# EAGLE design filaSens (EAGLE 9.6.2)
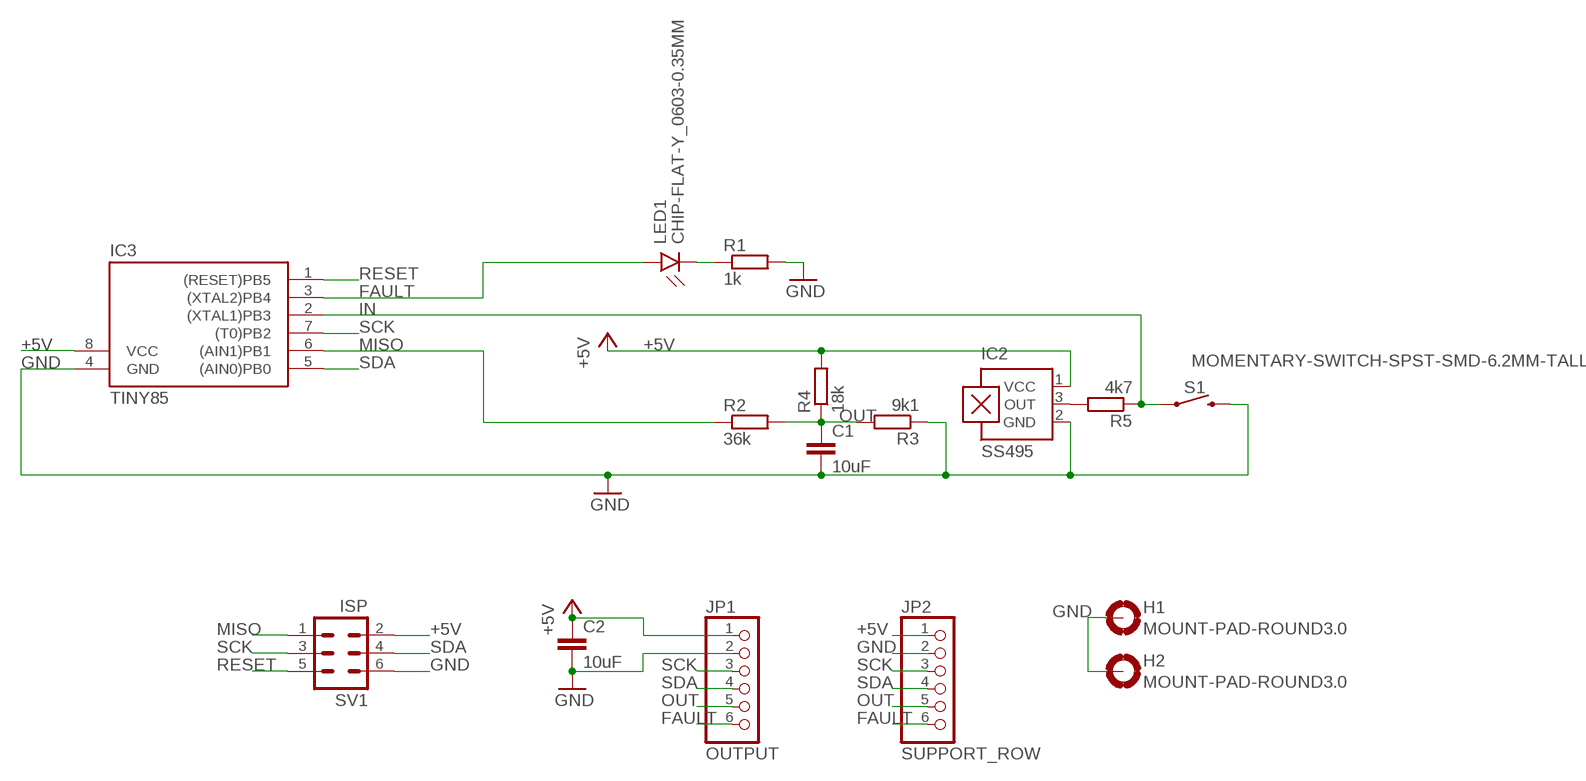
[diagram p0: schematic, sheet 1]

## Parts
C1  10uF  C-EUC0402  [C0402]
C2  10uF  C-EUC0402  [C0402]
H1  MOUNT-PAD-ROUND3.0  [3,0-PAD]
H2  MOUNT-PAD-ROUND3.0  [3,0-PAD]
IC2  SS495  A1302UA  [SIP3-UA]
IC3  TINY85  TINY10S  [SOIC8]
JP1  OUTPUT  PINHD-1X6  [1X06]
JP2  SUPPORT_ROW  PINHD-1X6  [1X06]
LED1  CHIP-FLAT-Y_0603-0.35MM  [LEDC1608X35N_FLAT-Y]
R1  1k  R-EU_R0402  [R0402]
R2  36k  R-EU_R0402  [R0402]
R3  9k1  R-EU_R0402  [R0402]
R4  18k  R-EU_R0402  [R0402]
R5  4k7  R-EU_R0402  [R0402]
S1  MOMENTARY-SWITCH-SPST-SMD-6.2MM-TALL  [TACTILE_SWITCH_SMD_6.2MM_TALL]
SV1  ISP  MA03-2  [MA03-2]

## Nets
+5V [power]: C2.1 IC2.1(VCC) IC3.8(VCC) JP1.1 JP2.1 R4.2 SV1.2
FAULT: IC3.3((XTAL2)PB4) JP1.6 JP2.6 LED1.A
GND [power]: C1.2 C2.2 H1.B3,0(MOUNT) H2.B3,0(MOUNT) IC2.2(GND) IC3.4(GND) JP1.2 JP2.2 R1.2 R3.1 S1.B2 SV1.6
IN: IC3.2((XTAL1)PB3) R5.1 S1.A2
MISO: IC3.6((AIN1)PB1) R2.1 SV1.1
N$1: IC2.3(OUT) R5.2
N$2: LED1.C R1.1
OUT: C1.1 JP1.5 JP2.5 R2.2 R3.2 R4.1
RESET: IC3.1((RESET)PB5) SV1.5
SCK: IC3.7((T0)PB2) JP1.3 JP2.3 SV1.3
SDA: IC3.5((AIN0)PB0) JP1.4 JP2.4 SV1.4

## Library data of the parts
C1 C2 = rcl:C-EU: CAPACITOR, European symbol; SPICEPREFIX: C
H1 H2 = holes:MOUNT-PAD-ROUND: MOUNTING PAD, round
IC2 = allegro:A13*?: Linear Hall Effect Sensor ICs Continuous-Time Ratiometric High-Temperature Operation Programmable Linear with Analog Output A1302 -Replacement- UGN3503 Source: http://www.allegromicro.com/en/Products/Part_Numbers/1301/1301.pdf http://www.allegromicro.com/en/Products/Part_Numbers/1321/1321.pdf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; MF: ALLEGRO MICROSYSTEMS, INC.; MPN: A1302EUA-T; OC_FARNELL: 1521708; OC_NEWARK: 31K6639
IC3 = atmel:TINY10: MICROCONTROLLER 1 Kbytes ROM; OC_FARNELL: unknown; OC_NEWARK: unknown
JP1 JP2 = pinhead:PINHD-1X6: PIN HEADER
LED1 = LED:CHIP-FLAT-Y; CATEGORY: LED; COLOR: YELLOW; DESCRIPTION: CHIP LED FLAT; SUB-CATEGORY: CHIP; TYPE: FLAT_TOP
R1-R5 = rcl:R-EU_: RESISTOR, European symbol; SPICEPREFIX: R
S1 = SparkFun-Switches:MOMENTARY-SWITCH-SPST: Momentary Switch (Pushbutton) - SPST; PROD_ID: SWCH-11966; SF_SKU: COM-12992
SV1 = con-lstb:MA03-2: PIN HEADER; OC_FARNELL: unknown; OC_NEWARK: unknown

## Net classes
0 default: width 0.254 mm
1 power: width 0.254 mm

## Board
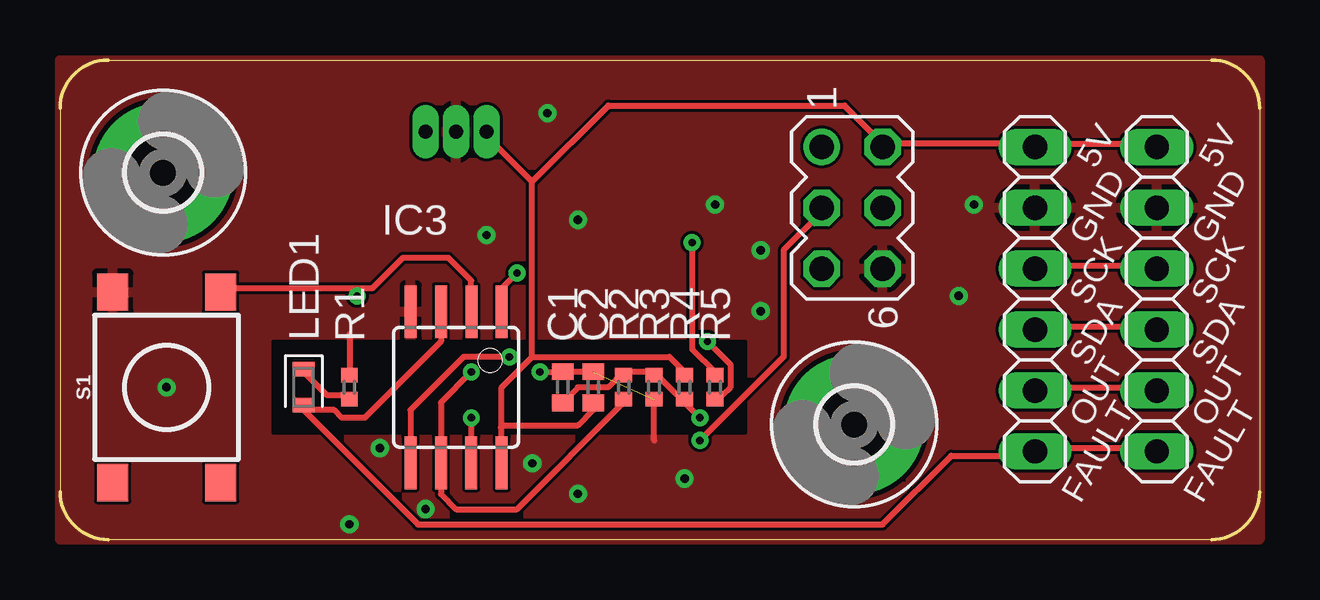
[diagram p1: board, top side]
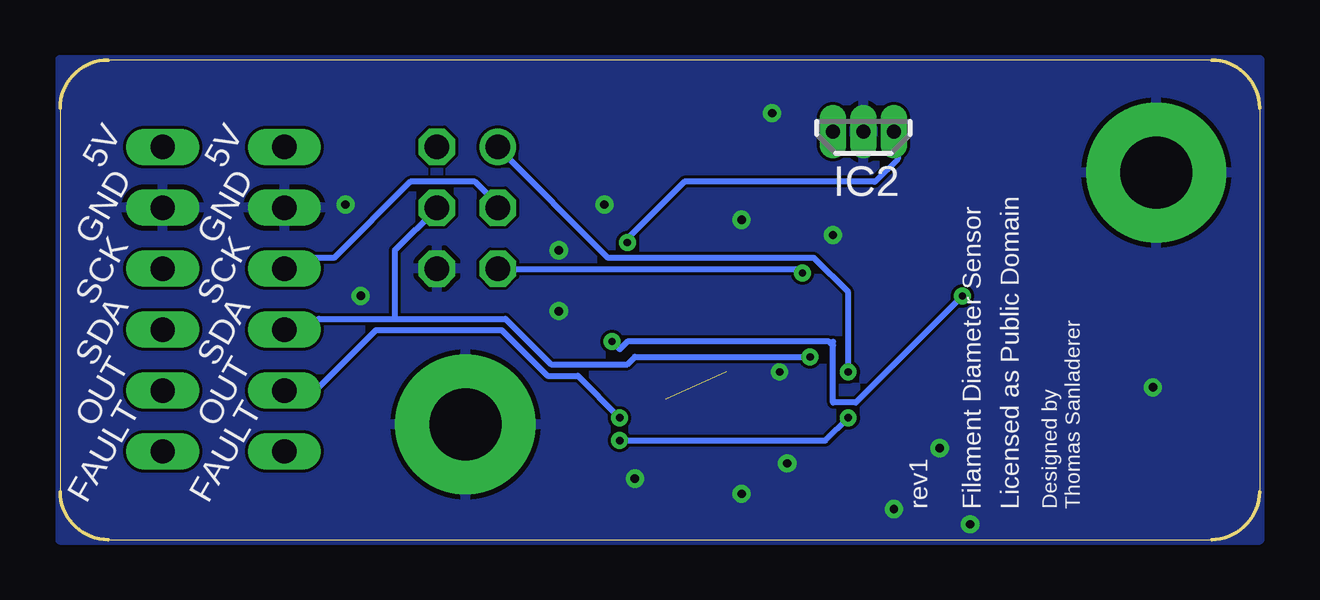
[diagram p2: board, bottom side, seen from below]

Size 50 x 20 mm. Coordinates in mm from the lower left corner, seen from the top.
Outline: 0,18 0,2 arc90 2,0 48,0 arc90 50,2 50,18 arc90 48,20 2,20 arc90 0,18
Copper layers (1*16): Top 0.035mm / dielectric 1.5mm / Bottom 0.035mm
Design rules "default *": minimum track width 10mil, minimum drill 0.3mm, track to track 5mil, track to pad 5mil, pad to pad 5mil, via to via 5mil, smd to smd 5mil, copper to edge 0mil, drill to drill 8mil, minimum pad ring 10mil, minimum via ring 8mil, stop-mask expansion 4mil, vias tented up to drill 28mil, thermal gap 8mil

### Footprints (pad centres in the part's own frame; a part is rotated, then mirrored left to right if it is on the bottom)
C0402 = smd 0.7 x 0.9: 1 -0.65,0; 2 0.65,0
3,0-PAD = drill 3 pad 5.842: B3,0 0,0
SIP3-UA = drill 0.6 pad 0.7 long: 1 -1.27,0; 2 0,0; 3 1.27,0
SOIC8 = smd 0.5 x 2.2: 1 -1.905,-3.154; 2 -0.645,-3.154; 3 0.625,-3.154; 4 1.895,-3.154; 5 1.905,3.154; 6 0.635,3.154; 7 -0.635,3.154; 8 -1.905,3.154
1X06 = drill 1.016 long: 1 -6.35,0; 2 -3.81,0; 3 -1.27,0; 4 1.27,0; 5 3.81,0; 6 6.35,0
LEDC1608X35N_FLAT-Y = smd 0.612 x 0.912: A 0.75,0; C -0.75,0
R0402 = smd 0.6 x 0.7: 1 -0.5,0; 2 0.5,0
TACTILE_SWITCH_SMD_6.2MM_TALL = smd 1.55 x 1.3: A1 -3.975,-2.25; A2 3.975,-2.25; B1 -3.975,2.25; B2 3.975,2.25
MA03-2 = drill 1.016: 1 -2.54,-1.27 | drill 1.016 octagon: 2 -2.54,1.27; 3 0,-1.27; 4 0,1.27; 5 2.54,-1.27; 6 2.54,1.27

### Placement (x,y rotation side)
C1  20.95,6.35 90 top
C2  22.23,6.35 90 top
H1  33.1,4.8 0 top
H2  4.3,15.3 0 top
IC2  16.51,17.01 0 bottom
IC3  16.51,6.35 180 top
JP1  40.64,10.03 270 top
JP2  45.72,10.03 270 top
LED1  10.16,6.35 270 top
R1  12.06,6.35 90 top
R2  23.5,6.35 90 top
R3  24.77,6.35 90 top
R4  26.04,6.35 90 top
R5  27.3,6.35 90 top
S1  4.45,6.35 90 top
SV1  33.02,13.84 270 top

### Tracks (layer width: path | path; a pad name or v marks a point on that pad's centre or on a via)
+5V
  Top 0.254: 40.64,16.51 34.29,16.51 | 40.64,16.51 45.72,16.51 JP2.1 | 40.64,16.51 JP1.1 | 19.68,7.62 25.4,7.62 26.04,6.99 R4.2 | 19.68,7.62 18.41,6.35 18.41,4.76 | 18.41,4.76 21.59,4.76 22.23,5.4 C2.1 | 19.68,14.92 17.78,16.83 IC2.1 | 19.68,7.62 19.68,14.92 | 34.29,16.51 32.7,18.1 22.86,18.1 19.68,14.92 | 34.29,16.51 SV1.2 | IC3.8 18.38,3.24 18.38,4.67 18.41,4.76
FAULT
  Top 0.254: JP2.6 45.72,3.81 40.64,3.81 JP1.6 40.64,3.49 37.15,3.49 34.29,0.64 14.92,0.64 10.16,5.4 | 10.16,5.4 11.43,5.4 11.75,5.08 12.7,5.08 15.88,8.26 15.88,9.21 IC3.3 | 10.16,5.4 LED1.A
GND  (via drill 0.3, 0.35)  (1 unrouted)
  Top 0.254: 20.95,6.99 22.23,6.99 C2.2 | 24.77,4.13 R3.1 | v20,6.99 20.95,6.99 | 20.95,6.99 C1.2 | 12.06,8.57 R1.2
  other vias: 21.59,13.34 27.3,13.97 29.21,12.06 37.47,10.16 38.1,13.97 4.45,6.35 13.34,3.81 19.68,3.17 21.59,1.91 26.04,2.54 29.21,9.53 15.24,1.27 12.06,0.64 17.78,12.7 20.32,17.78
  pour Bottom: 0,20 50,20 50,0 0,0
  pour Top (rank 3): 0,20 50,20 50,0 0,0
  cutout Top (rank 2): 8.89,4.45 8.89,8.26 28.57,8.26 28.57,4.45
IN  (via drill 0.3)
  Top 0.254: v26.99,8.26 27.94,7.3 27.94,6.35 27.62,6.03 27.3,6.03 R5.1 | 12.38,10.48 13.02,10.48 14.29,11.75 16.19,11.75 17.14,10.79 17.14,9.53 IC3.2 | 12.38,10.48 6.99,10.48 S1.A2 | 12.38,10.48 v12.38,10.16
  Bottom 0.254: 17.78,8.1 17.86,8.18 | 17.86,8.18 17.94,8.26 26.35,8.26 26.67,7.94 v26.99,8.26 | v12.38,10.16 16.83,5.71 17.78,5.71 17.78,8.26 17.86,8.18
MISO  (via drill 0.3)
  Top 0.254: R2.1 23.5,5.71 19.05,1.27 16.51,1.27 15.88,1.91 IC3.6 15.88,5.71 v17.14,6.99
  Bottom 0.254: 17.14,6.83 v17.14,6.99 17.14,10.32 18.57,11.75 27.15,11.75 31.75,16.35 SV1.1
N$1  (via drill 0.3)
  Top 0.254: v26.35,12.38 26.35,7.94 27.3,6.99 R5.2
  Bottom 0.254: 26.43,12.46 23.97,14.92 16.03,14.92 15.08,15.88 15.08,16.99 15.24,16.99 IC2.3 | 26.43,12.46 26.51,12.38 | v26.35,12.38 26.43,12.46
N$2
  Top 0.254: R1.1 12.06,6.03 11.11,6.03 10.16,6.99 LED1.C
OUT  (via drill 0.3)
  Top 0.254: 24.77,6.99 23.5,6.99 | 24.77,6.99 25.72,6.03 26.04,6.03 R4.1 26.04,5.71 v26.67,5.08 | 24.77,6.99 R3.2 | 23.5,6.99 22.86,6.35 21.59,6.35 20.95,5.71 C1.1 | 23.5,6.99 R2.2 | JP2.5 45.72,6.35 40.64,6.35 JP1.5
  Bottom 0.254: v26.67,5.08 28.42,6.83 29.69,6.83 31.59,8.73 36.83,8.73 39.21,6.35 40.64,6.35 JP1.5
RESET  (via drill 0.3)
  Top 0.254: IC3.1 18.41,10.48 v19.05,11.11
  Bottom 0.254: 18.97,11.19 19.05,11.27 31.75,11.27 SV1.5 | 18.97,11.19 18.89,11.11 | v19.05,11.11 18.97,11.19
SCK  (via drill 0.3)
  Top 0.254: v17.14,5.08 IC3.7 | v26.67,4.13 30.16,7.62 30.16,12.06 31.75,13.65 SV1.3 | JP2.3 45.72,11.43 40.64,11.43 JP1.3
  Bottom 0.254: JP1.3 40.64,11.43 40.32,11.75 38.58,11.75 35.4,14.92 32.7,14.92 31.75,13.97 SV1.3 | v17.14,5.08 18.1,4.13 v26.67,4.13
SDA  (via drill 0.3)
  Top 0.254: IC3.5 14.61,5.4 16.83,7.62 v18.73,7.62 | JP2.4 45.72,8.89 40.64,8.89 JP1.4
  Bottom 0.254: 18.57,7.46 v18.73,7.62 26.04,7.62 26.35,7.3 29.53,7.3 31.43,9.21 36.04,9.21 | 36.04,9.21 39.21,9.21 39.53,8.89 40.64,8.89 JP1.4 | 36.04,9.21 36.04,12.06 34.29,13.81 SV1.4

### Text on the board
tNames: 5V | 5V | GND | GND | SCK | SCK | SDA | SDA | OUT | OUT | FAULT | FAULT
bNames: 5V | 5V | GND | GND | SCK | SCK | SDA | SDA | OUT | OUT | Designed by / Thomas Sanladerer | Licensed as Public Domain | Filament Diameter Sensor | rev1 | FAULT | FAULT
